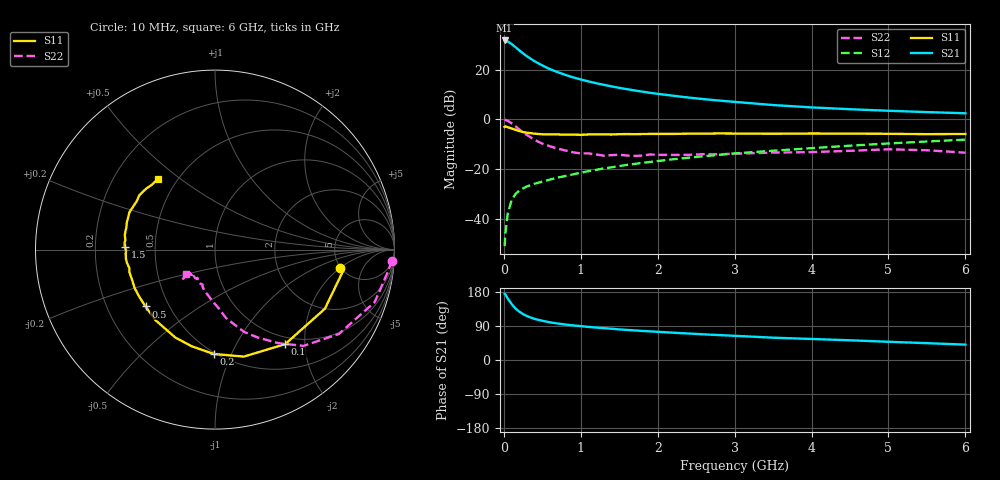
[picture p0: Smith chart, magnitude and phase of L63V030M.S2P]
!  INFINEON TECHNOLOGIES Small Signal Semiconductors
! BFR380L3 , Si-NPN RF-Transistor in TSLP-3-1
!  Vce=3 V,  Ic=30 mA
! Common Emitter S-Parameters:  07. March 2005
#  GHz  S  MA  R  50
! f  S11  S21  S12  S22
! GHz  Mag  Ang  Mag  Ang  Mag  Ang  Mag  Ang
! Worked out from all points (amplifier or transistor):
!   36 points, 10 MHz to 6 GHz, reference 50 ohm
!   highest |S21| = 31.8 dB at 10 MHz (marker M1)
!   |S21| within 3 dB of that: start of sweep to 163 MHz
!   unconditionally stable (mu >= 1): 1.683 GHz to 4.813 GHz
!   at 250 MHz: K = 0.43, MSG = 27.2 dB, |S12| = -27.8 dB
!   at 1.4 GHz: K = 0.97, MSG = 16.3 dB, |S12| = -19.3 dB
!   at 6 GHz: K = 0.98, MSG = 5.3 dB, |S12| = -8.2 dB
!   S11 on the Smith chart (normalised r, x): 10 MHz: 4.94, -2.00; 100 MHz: 0.88, -1.63; 200 MHz: 0.49, -0.86; 500 MHz: 0.37, -0.31; 1.5 GHz: 0.33, +0.01; 6 GHz: 0.39, +0.42
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0.01  0.7049 -8.3  38.72 174.5  0.0028 76.8  0.9884 -3.6
0.02  0.7251 -9.0  38.23 173.0  0.005 85.3  0.9703 -7.5
0.05  0.6952 -28.3  36.91 162.6  0.0124 80.1  0.9367 -18.2
0.1  0.656 -53.4  32.87 148.0  0.0236 68.6  0.8354 -34.2
0.15  0.6175 -74.9  28.51 136.2  0.0313 61.2  0.7287 -47.4
0.2  0.5813 -90.8  24.51 127.6  0.0366 57.0  0.6297 -55.9
0.25  0.5541 -103.5  21.3 121.2  0.0408 54.1  0.5424 -64.3
0.3  0.5377 -114.2  18.57 115.9  0.0445 53.7  0.4856 -70.6
0.4  0.5145 -130.0  14.77 108.5  0.0506 53.4  0.3856 -80.9
0.5  0.5003 -140.7  12.15 103.5  0.0558 54.3  0.3244 -86.8
0.6  0.4969 -148.6  10.25 99.4  0.0613 55.7  0.2868 -93.0
0.7  0.4964 -154.4  8.906 96.3  0.0673 56.9  0.2566 -98.8
0.8  0.4915 -160.3  7.854 93.6  0.0725 58.4  0.2368 -104.5
0.9  0.4932 -165.2  7.001 91.3  0.0781 59.6  0.2167 -108.7
1.1  0.496 -171.3  5.801 87.3  0.0907 61.3  0.2068 -114.5
1.5  0.5027 178.2  4.31 80.8  0.1147 63.7  0.1935 -124.6
1.8  0.5062 172.0  3.616 76.7  0.133 64.5  0.1864 -129.9
2.2  0.5091 165.8  2.986 72.0  0.1571 64.9  0.1919 -133.0
3.5  0.5128 148.1  1.94 58.9  0.2335 63.1  0.2142 -138.4
4.5  0.5162 141.9  1.598 52.0  0.2953 61.7  0.2326 -137.9
5.5  0.5036 133.9  1.399 44.4  0.3579 58.2  0.2386 -137.5
6  0.5076 128.8  1.325 40.6  0.3908 55.9  0.2131 -139.5
